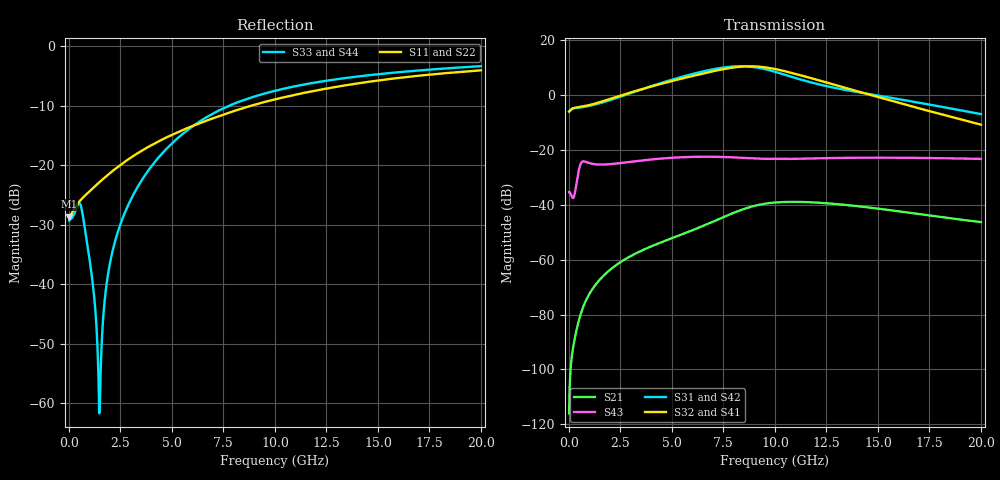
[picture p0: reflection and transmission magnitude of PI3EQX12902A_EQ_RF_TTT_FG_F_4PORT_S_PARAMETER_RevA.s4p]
! NPort=4 DATA=2000 NOISE=0 GROUPDELAY=0 COMPLEX_DATAFORMAT=POLAR
! NumOfBlock=1 NumOfParam=0
! .MODEL Smodel S TSTONEFILE=PI3EQX12902A_EQ_RF_TTT_FG_F_4PORT_S_PARAMETER_RevA.s4p TYPE=S
!  -- The above .MODEL line can be used for the S element in the netlist.
! The s parameter is extracted from the linear redriver, it is not bi-directional; only s(4,1)s(4,2) and s(3,1)s(3,2)
! should be the insertion loss
!Port definition:
!Port1 = input+
!Port2 = input-
!Port3 = output+
!Port4 = output-
# Hz S MA R  50
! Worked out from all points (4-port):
!   2000 points, 10 MHz to 20 GHz, reference 50 ohm
!   strongest paths, dB at 10 MHz, 5.01 GHz, 10.01 GHz, 15.01 GHz, 20 GHz:
!     S32: -6.0, 5.1, 9.4, -0.8, -10.8
!     S41: -6.0, 5.0, 9.3, -0.8, -10.8
!     S31: -6.0, 5.6, 8.4, -0.2, -7.0
!     S42: -6.0, 5.5, 8.2, -0.4, -7.1
!     S43: -35.3, -22.9, -23.3, -22.9, -23.3
!     S21: -116.0, -52.2, -39.2, -41.4, -46.3
!   lowest |S11| = -28.6 dB at 10 MHz (marker M1), VSWR 1.08, Z = 46.4 - j0.0607 ohm
!   |S11| at or under -10 dB: start of sweep to 8.846 GHz
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1e7  0.03704 -179.0  1.589e-06 51.9  0 0.0  0 0.0
     1.589e-06 51.9  0.03704 -179.0  0 0.0  0 0.0
     0.4994 0.9  0.4994 -179.1  0.03429 6.0  0.01709 -177.1
     0.4994 -179.1  0.4994 0.9  0.01709 -177.1  0.03429 6.0
5.96e9  0.212 -112.1  0.00339 92.2  1.61e-06 -23.0  1.02e-06 87.5
        0.003386 92.2  0.212 -112.1  1.021e-06 87.7  1.602e-06 -22.7
        2.386 -45.8  2.197 111.2  0.2098 -46.2  0.07397 145.0
        2.187 111.2  2.349 -46.4  0.07436 145.2  0.2092 -46.2
7.74e9  0.2751 -111.8  0.006504 76.8  5.859e-06 -76.4  3.814e-06 43.7
        0.006485 76.8  0.2751 -111.8  3.813e-06 43.8  5.83e-06 -75.9
        3.241 -95.6  3.062 60.2  0.3141 -63.8  0.073 126.2
        3.039 60.2  3.178 -96.0  0.07348 126.2  0.3134 -63.7
9.21e9  0.3296 -113.2  0.009977 48.1  1.116e-05 -123.6  8.732e-06 -7.3
        0.009936 48.2  0.3296 -113.2  8.704e-06 -7.2  1.113e-05 -122.8
        3.121 -145.5  3.274 6.6  0.3869 -75.8  0.06871 115.0
        3.239 6.7  3.051 -145.8  0.06915 114.8  0.3865 -75.6
1.091e10  0.3884 -115.8  0.01134 11.6  1.626e-05 -165.1  1.409e-05 -67.2
          0.0113 11.9  0.3884 -115.8  1.399e-05 -67.0  1.633e-05 -164.2
          2.082 169.4  2.467 -51.0  0.4577 -86.8  0.06827 106.0
          2.436 -50.6  2.028 169.5  0.06853 105.6  0.4578 -86.7
1.347e10  0.471 -120.1  0.009888 -28.1  2.581e-05 148.7  1.842e-05 -137.8
          0.009883 -27.5  0.4711 -120.1  1.822e-05 -137.4  2.61e-05 149.3
          1.225 129.8  1.33 -114.8  0.541 -99.6  0.07149 89.1
          1.317 -114.0  1.196 130.5  0.07147 88.8  0.5415 -99.5
2e10  0.6267 -131.6  0.004751 -72.9  4.268e-05 50.3  1.771e-05 102.1
      0.004838 -72.7  0.6267 -131.6  1.746e-05 103.5  4.329e-05 50.4
      0.4476 41.7  0.2877 134.8  0.6794 -119.6  0.06845 46.2
      0.2883 135.9  0.4434 42.6  0.06837 46.1  0.6797 -119.6
